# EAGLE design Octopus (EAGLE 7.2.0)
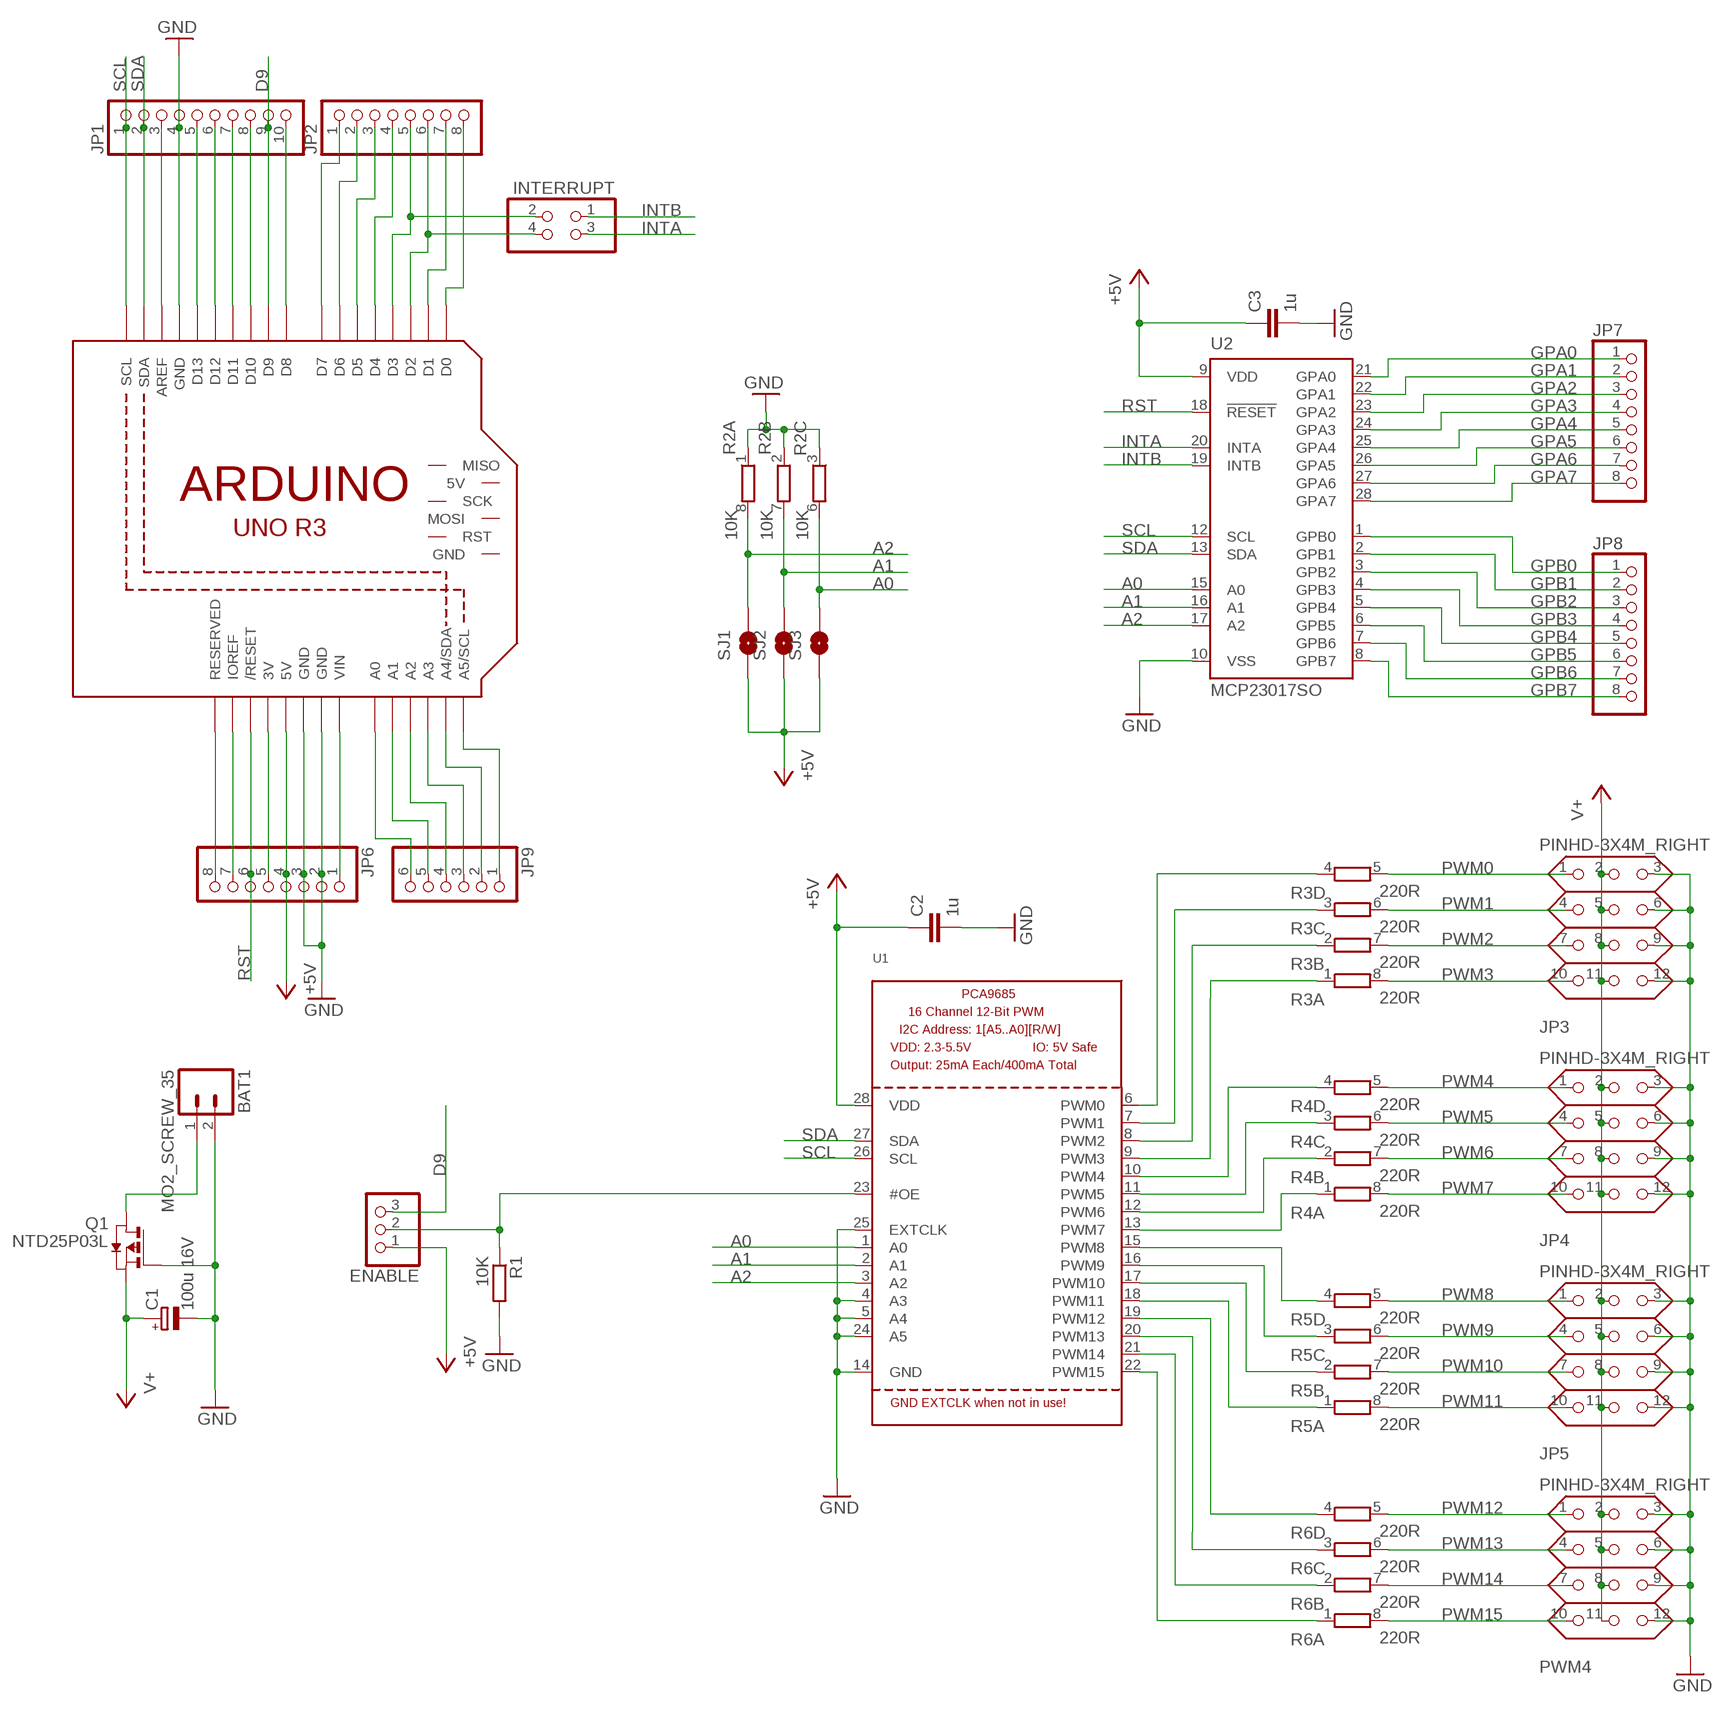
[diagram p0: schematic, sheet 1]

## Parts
BAT1  MO2_SCREW_35  [SCREWTERMINAL-3.5MM-2-NS]
C1  100u 16V  CPOLPANASONIC_E  [PANASONIC_E]
C2  1u  C0805  [C0805]
C3  1u  C0805  [C0805]
ENABLE  PINHD-1X3  [1X03M]
INTERRUPT  PINHD-2X2  [2X02M]
JP1  PINHD-1X10F_LONG  [1X10F_LONG]
JP2  PINHD-1X8F_LONG  [1X08F_LONG]
JP3  PINHD-3X4M_RIGHT  [3X04M_RIGHT]
JP4  PINHD-3X4M_RIGHT  [3X04M_RIGHT]
JP5  PINHD-3X4M_RIGHT  [3X04M_RIGHT]
JP6  PINHD-1X8F_LONG  [1X08F_LONG]
JP7  PINHD-1X81X08M_RIGHT  [1X08M_RIGHT]
JP8  PINHD-1X81X08M_RIGHT  [1X08M_RIGHT]
JP9  PINHD-1X6F_LONG  [1X06F_LONG]
M1  ARDUINO_R3_ICSP  [ARDUINOR3_ICSP]
PWM4  PINHD-3X4M_RIGHT  [3X04M_RIGHT]
Q1  NTD25P03L  [DPACK_2]
R1  10K  R0805  [R0805]
R2  10K  RESISTOR-ARRAY0603-ARV  [R0603X4]
R3  220R  RESISTOR-ARRAY0603-ARV  [R0603X4]
R4  220R  RESISTOR-ARRAY0603-ARV  [R0603X4]
R5  220R  RESISTOR-ARRAY0603-ARV  [R0603X4]
R6  220R  RESISTOR-ARRAY0603-ARV  [R0603X4]
SJ1  JUMPER-PAD-2-NOYES_SILK  [PAD-JUMPER-2-NO_YES_SILK]
SJ2  JUMPER-PAD-2-NOYES_SILK  [PAD-JUMPER-2-NO_YES_SILK]
SJ3  JUMPER-PAD-2-NOYES_SILK  [PAD-JUMPER-2-NO_YES_SILK]
U1  PCA9685  [TSSOP28]
U2  MCP23017SO  [SO28W]

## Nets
+5V: C2.1 C3.1 ENABLE.1 JP6.4 M1.5V SJ1.1 SJ2.1 SJ3.1 U1.28(VDD) U2.9(VDD)
A0: R2.6 SJ3.2 U1.1(A0) U2.15(A0)
A1: R2.7 SJ2.2 U1.2(A1) U2.16(A1)
A2: R2.8 SJ1.2 U1.3(A2) U2.17(A2)
D9: ENABLE.3 JP1.9 M1.D9
GND: BAT1.2 C1.- C2.2 C3.2 JP1.4 JP3.3 JP3.6 JP3.9 JP3.12 JP4.3 JP4.6 JP4.9 JP4.12 JP5.3 JP5.6 JP5.9 JP5.12 JP6.2 JP6.3 M1.GND M1.GND@1(GND) M1.GND@2(GND) PWM4.3 PWM4.6 PWM4.9 PWM4.12 Q1.G R1.2 R2.1 R2.2 R2.3 U1.4(A3) U1.5(A4) U1.14(GND) U1.24(A5) U1.25(EXTCLK) U2.10(VSS)
GPA0: JP7.1 U2.21(GPA0)
GPA1: JP7.2 U2.22(GPA1)
GPA2: JP7.3 U2.23(GPA2)
GPA3: JP7.4 U2.24(GPA3)
GPA4: JP7.5 U2.25(GPA4)
GPA5: JP7.6 U2.26(GPA5)
GPA6: JP7.7 U2.27(GPA6)
GPA7: JP7.8 U2.28(GPA7)
GPB0: JP8.1 U2.1(GPB0)
GPB1: JP8.2 U2.2(GPB1)
GPB2: JP8.3 U2.3(GPB2)
GPB3: JP8.4 U2.4(GPB3)
GPB4: JP8.5 U2.5(GPB4)
GPB5: JP8.6 U2.6(GPB5)
GPB6: JP8.7 U2.7(GPB6)
GPB7: JP8.8 U2.8(GPB7)
INTA: INTERRUPT.3 U2.20(INTA)
INTB: INTERRUPT.1 U2.19(INTB)
N$1: R3.4 U1.6(PWM0)
N$2: R3.3 U1.7(PWM1)
N$3: R3.2 U1.8(PWM2)
N$4: R3.1 U1.9(PWM3)
N$5: R4.4 U1.10(PWM4)
N$6: R4.3 U1.11(PWM5)
N$7: R4.2 U1.12(PWM6)
N$8: R4.1 U1.13(PWM7)
N$9: R5.4 U1.15(PWM8)
N$10: R5.3 U1.16(PWM9)
N$11: R5.2 U1.17(PWM10)
N$12: R5.1 U1.18(PWM11)
N$13: R6.4 U1.19(PWM12)
N$14: R6.3 U1.20(PWM13)
N$15: R6.2 U1.21(PWM14)
N$16: R6.1 U1.22(PWM15)
N$17: JP1.3 M1.AREF
N$18: JP1.5 M1.D13
N$19: BAT1.1 Q1.D
N$20: JP1.6 M1.D12
N$21: JP1.7 M1.D11
N$22: JP1.8 M1.D10
N$23: JP1.10 M1.D8
N$24: JP2.1 M1.D7
N$25: JP2.2 M1.D6
N$26: JP2.3 M1.D5
N$27: JP2.4 M1.D4
N$28: JP2.7 M1.D1
N$29: JP2.8 M1.D0
N$30: JP6.8 M1.RESERVED
N$31: JP6.7 M1.IOREF
N$32: JP6.5 M1.3V
N$33: JP6.1 M1.VIN
N$34: INTERRUPT.2 JP2.5 M1.D3
N$35: JP9.6 M1.A0
N$36: JP9.5 M1.A1
N$37: JP9.4 M1.A2
N$38: JP9.3 M1.A3
N$39: JP9.2 M1.A4(A4/SDA)
N$40: JP9.1 M1.A5(A5/SCL)
N$41: INTERRUPT.4 JP2.6 M1.D2
N$42: ENABLE.2 R1.1 U1.23(#OE)
PWM0: JP3.1 R3.5
PWM1: JP3.4 R3.6
PWM2: JP3.7 R3.7
PWM3: JP3.10 R3.8
PWM4: JP4.1 R4.5
PWM5: JP4.4 R4.6
PWM6: JP4.7 R4.7
PWM7: JP4.10 R4.8
PWM8: JP5.1 R5.5
PWM9: JP5.4 R5.6
PWM10: JP5.7 R5.7
PWM11: JP5.10 R5.8
PWM12: PWM4.1 R6.5
PWM13: PWM4.4 R6.6
PWM14: PWM4.7 R6.7
PWM15: PWM4.10 R6.8
RST: JP6.6 M1.RESET(/RESET) U2.18(!RESET)
SCL: JP1.1 M1.SCL U1.26(SCL) U2.12(SCL)
SDA: JP1.2 M1.SDA U1.27(SDA) U2.13(SDA)
V+: C1.+ JP3.2 JP3.5 JP3.8 JP3.11 JP4.2 JP4.5 JP4.8 JP4.11 JP5.2 JP5.5 JP5.8 JP5.11 PWM4.2 PWM4.5 PWM4.8 PWM4.11 Q1.S
Unconnected: M1.5V_ICSP(5V) M1.GND@3(GND) M1.MISO M1.MOSI M1.RESET_ICSP(RST) M1.SCK R2.4 R2.5

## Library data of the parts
BAT1 = Max-Connectors:MO2_SCREW_35
C1 = Max-RCL:CPOL
C2 C3 = Max-RCL:C
ENABLE = Max-PinHead:PINHD-1X3: PIN HEADER
INTERRUPT = Max-PinHead:PINHD-2X2
JP1 = Max-PinHead:PINHD-1X10: PIN HEADER
JP2 JP6-JP8 = Max-PinHead:PINHD-1X8: PIN HEADER
JP3-JP5 PWM4 = Max-PinHead:PINHD-3X4
JP9 = Max-PinHead:PINHD-1X6: PIN HEADER
M1 = Max-Arduino:ARDUINO_R3_ICSP
Q1 = Max-Mosfets:NTD25P03L
R1 = Max-RCL:R
R2-R6 = Max-RCL:RESISTOR-ARRAY: Array Chip Resistor Source: RS Component / Phycomp
SJ1-SJ3 = Max-Connectors:JUMPER-PAD-2-NO
U1 = Max-IOExpanders:PCA9685: PCA9685 - 16 Channel 12-Bit I2C PWM Controller 5.0V tolerant 16 channel, 12-bit I2C PWM controller with 25mA per output (max. 400mA total) Digikey: 568-5931-1-ND
U2 = Max-IOExpanders:MCP23017: http://ww1.microchip.com/downloads/en/DeviceDoc/21952a.pdf Source: http://ww1.microchip.com/downloads/en/DeviceDoc/21952a.pdf

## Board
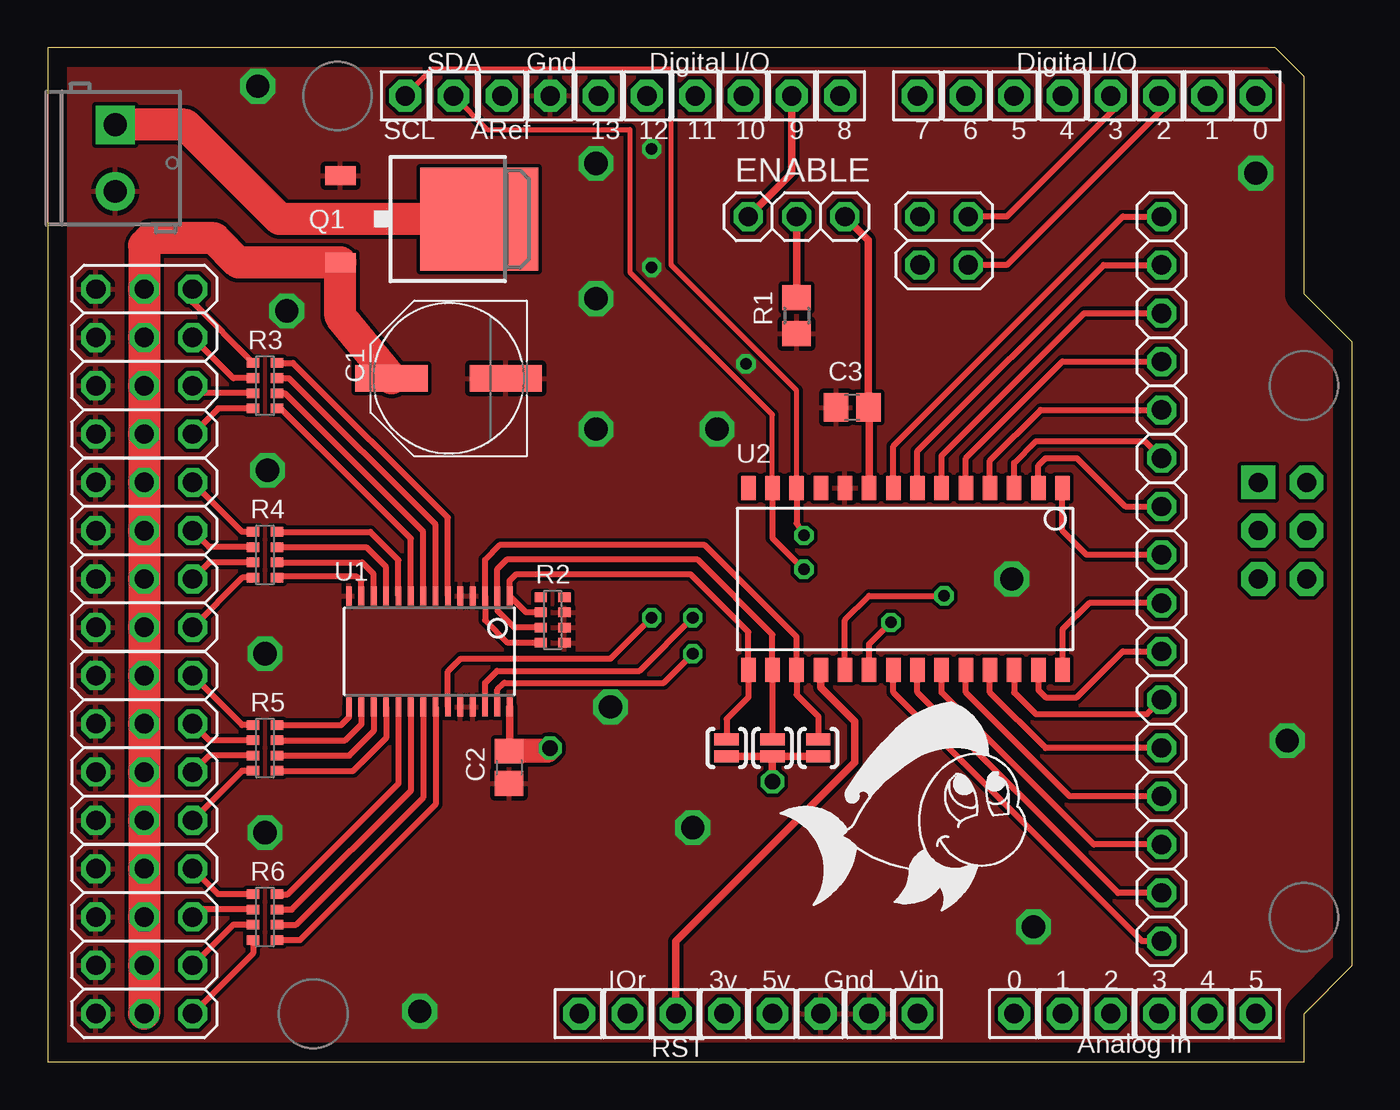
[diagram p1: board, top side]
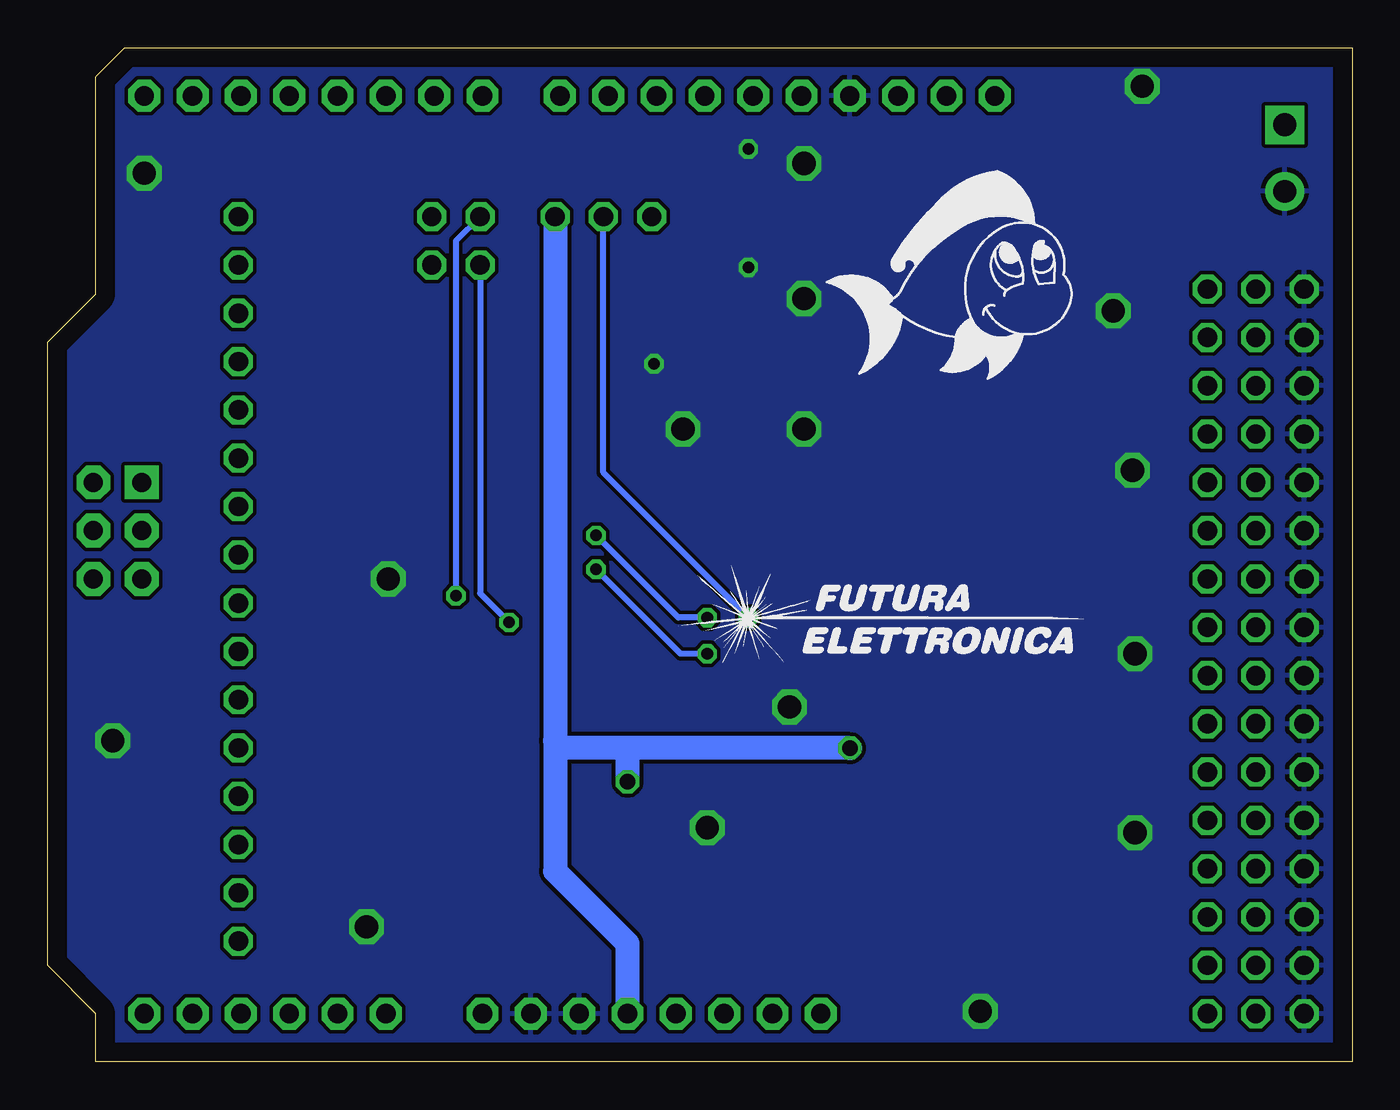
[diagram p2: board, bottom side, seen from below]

Size 68.58 x 53.34 mm. Coordinates in mm from the lower left corner, seen from the top.
Copper layers (1*16): Top 0.035mm / dielectric 1.5mm / Bottom 0.035mm
Design rules "default": minimum track width 10mil, minimum drill 24mil, track to track 8mil, track to pad 8mil, pad to pad 8mil, via to via 8mil, smd to smd 8mil, copper to edge 40mil, drill to drill 8mil, minimum pad ring 10mil, minimum via ring 8mil, stop-mask expansion 4mil, vias tented up to drill 0mil, thermal gap 10mil

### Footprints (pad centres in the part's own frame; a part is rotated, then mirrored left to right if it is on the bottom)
SCREWTERMINAL-3.5MM-2-NS = drill 1.2 pad 2.032 square: 1 -1.778,0 | drill 1.2 pad 2.032: 2 1.722,0
PANASONIC_E = smd 3.8 x 1.4: + 3,0; - -3,0
C0805 = smd 1.3 x 1.5: 1 -0.85,0; 2 0.85,0
1X03M = drill 1.016 octagon: 1 -2.54,0; 2 0,0; 3 2.54,0
2X02M = drill 1.016 octagon: 1 -1.27,-1.27; 2 -1.27,1.27; 3 1.27,-1.27; 4 1.27,1.27
1X10F_LONG = drill 1.016 octagon: 1 -11.43,0; 2 -8.89,0; 3 -6.35,0; 4 -3.81,0; 5 -1.27,0; 6 1.27,0; 7 3.81,0; 8 6.35,0; 9 8.89,0; 10 11.43,0
1X08F_LONG = drill 1.016 octagon: 1 -8.89,0; 2 -6.35,0; 3 -3.81,0; 4 -1.27,0; 5 1.27,0; 6 3.81,0; 7 6.35,0; 8 8.89,0
3X04M_RIGHT = drill 1.016 octagon: 1 -2.54,-3.81; 2 0,-3.81; 3 2.54,-3.81; 4 -2.54,-1.27; 5 0,-1.27; 6 2.54,-1.27; 7 -2.54,1.27; 8 0,1.27; 9 2.54,1.27; 10 -2.54,3.81; 11 0,3.81; 12 2.54,3.81
1X08M_RIGHT = drill 1.016 octagon: 1 -8.89,0; 2 -6.35,0; 3 -3.81,0; 4 -1.27,0; 5 1.27,0; 6 3.81,0; 7 6.35,0; 8 8.89,0
1X06F_LONG = drill 1.016 octagon: 1 -6.35,0; 2 -3.81,0; 3 -1.27,0; 4 1.27,0; 5 3.81,0; 6 6.35,0
ARDUINOR3_ICSP = drill 1 pad 1.676 octagon: 3V 35.56,2.54; 5V 38.1,2.54; A0 50.8,2.54; A1 53.34,2.54; A2 55.88,2.54; A3 58.42,2.54; A4 60.96,2.54; A5 63.5,2.54; AREF 23.876,50.8; D0 63.5,50.8; D1 60.96,50.8; D2 58.42,50.8; D3 55.88,50.8; D4 53.34,50.8; D5 50.8,50.8; D6 48.26,50.8; D7 45.72,50.8; D8 41.656,50.8; D9 39.116,50.8; D10 36.576,50.8; D11 34.036,50.8; D12 31.496,50.8; D13 28.956,50.8; GND 26.416,50.8; GND@1 43.18,2.54; GND@2 40.64,2.54; IOREF 30.48,2.54; RESERVED 27.94,2.54; RESET 33.02,2.54; SCL 18.796,50.8; SDA 21.336,50.8; VIN 45.72,2.54 | drill 1 pad 1.778 octagon: 5V_ICSP 66.167,30.48; GND@3 66.167,25.4; MOSI 66.167,27.94; RESET_ICSP 63.627,25.4; SCK 63.627,27.94 | drill 1 pad 1.778 square: MISO 63.627,30.48
DPACK_2 = smd 5.4 x 6.2: D 0,2.5 | smd 1 x 1.6: G -2.28,-4.8; S 2.28,-4.8
R0805 = smd 1.3 x 1.5: 1 -0.95,0; 2 0.95,0
R0603X4 = smd 0.5 x 0.65: 1 -1.2,-0.625; 2 -0.4,-0.625; 3 0.4,-0.625; 4 1.2,-0.625; 5 1.2,0.625; 6 0.4,0.625; 7 -0.4,0.625; 8 -1.2,0.625
PAD-JUMPER-2-NO_YES_SILK = smd 0.635 x 1.27: 1 -0.45,0; 2 0.45,0
TSSOP28 = smd 0.305 x 0.991: 1 -4.225,-2.918; 2 -3.575,-2.918; 3 -2.925,-2.918; 4 -2.275,-2.918; 5 -1.625,-2.918; 6 -0.975,-2.918; 7 -0.325,-2.918; 8 0.325,-2.918; 9 0.975,-2.918; 10 1.625,-2.918; 11 2.275,-2.918; 12 2.925,-2.918; 13 3.575,-2.918; 14 4.225,-2.918; 15 4.225,2.918; 16 3.575,2.918; 17 2.925,2.918; 18 2.275,2.918; 19 1.625,2.918; 20 0.975,2.918; 21 0.325,2.918; 22 -0.325,2.918; 23 -0.975,2.918; 24 -1.625,2.918; 25 -2.275,2.918; 26 -2.925,2.918; 27 -3.575,2.918; 28 -4.225,2.918
SO28W = smd 0.762 x 1.27: 1 -7.62,-4.78; 2 -6.35,-4.78; 3 -5.08,-4.78; 4 -3.81,-4.78; 5 -2.54,-4.78; 6 -1.27,-4.78; 7 0,-4.78; 8 1.27,-4.78; 9 2.54,-4.78; 10 3.81,-4.78; 11 5.08,-4.78; 12 6.35,-4.78; 13 7.62,-4.78; 14 8.89,-4.78; 15 8.89,4.78; 16 7.62,4.78; 17 6.35,4.78; 18 5.08,4.78; 19 3.81,4.78; 20 2.54,4.78; 21 1.27,4.78; 22 0,4.78; 23 -1.27,4.78; 24 -2.54,4.78; 25 -3.81,4.78; 26 -5.08,4.78; 27 -6.35,4.78; 28 -7.62,4.78

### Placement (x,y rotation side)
BAT1  3.56,47.5 270 top
C1  21.08,35.94 180 top
C2  24.26,15.49 270 top
C3  42.29,34.42 180 top
ENABLE  39.37,44.45 180 top
INTERRUPT  47.12,43.18 270 top
JP1  30.23,50.8 0 top
JP2  54.61,50.8 0 top
JP3  5.08,36.83 180 top
JP4  5.08,26.67 180 top
JP5  5.08,16.51 180 top
JP6  36.83,2.54 180 top
JP7  58.55,15.24 90 top
JP8  58.55,35.56 90 top
JP9  57.15,2.54 180 top
M1  0,0 0 top
PWM4  5.08,6.35 180 top
Q1  20.19,44.32 270 top
R1  39.37,39.24 270 top
R2  26.54,23.24 90 top
R3  11.43,35.56 90 top
R4  11.43,26.67 90 top
R5  11.43,16.51 90 top
R6  11.43,7.62 90 top
SJ1  40.51,16.51 90 top
SJ2  38.1,16.51 90 top
SJ3  35.69,16.51 90 top
U1  20.07,21.59 180 top
U2  45.72,25.4 180 top
U$1  [FISHINO]  40.26,8.26 0 top
U$2  [FISHINO]  25.91,36.2 0 bottom
U$4  [FUTURA]  35.43,20.95 0 bottom

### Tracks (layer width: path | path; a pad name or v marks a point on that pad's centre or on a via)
+5V  (via drill 0.81)
  Top 0.406: U1.28 24.29,16.38 C2.1 | U2.9 43.18,34.38 C3.1 43.14,43.22 ENABLE.1 | SJ2.1 SJ1.1 | SJ3.1 SJ2.1 | SJ2.1 v38.1,14.73
  Top 1.27: 24.29,16.38 26.28,16.38 v26.42,16.51
  Bottom 1.27: JP6.4 38.1,6.22 41.91,10.03 41.91,16.89 | v26.42,16.51 38.1,16.51 | 38.1,16.51 41.53,16.51 41.91,16.89 | ENABLE.1 41.91,16.89 | v38.1,14.73 38.1,16.51
A0
  Top 0.305: SJ3.2 35.69,18.03 36.83,19.18 U2.15 36.83,22.61 33.78,25.65 24.64,25.65 24.29,25.31 U1.1 25.16,23.64 R2.6
A1
  Top 0.305: R2.7 24.53,22.84 23.64,23.73 U1.2 23.64,25.93 24.13,26.42 34.16,26.42 38.1,22.48 U2.16 SJ2.2
A2
  Top 0.305: R2.8 24.19,22.04 22.99,23.24 U1.3 22.99,26.42 23.75,27.18 34.54,27.18 39.37,22.35 U2.17 39.37,19.3 40.51,18.16 SJ1.2
D9
  Top 0.406: ENABLE.3 39.12,46.74 JP1.9
GND  (via drill 0.61, 1.22)
  other vias: 11.43,12.06 11.43,21.46 11.56,31.11 12.57,39.5 35.18,33.27 28.83,33.27 19.56,2.67 33.91,12.32 29.59,18.67 50.67,25.4 28.83,47.24 28.83,40.13 11.05,51.31 51.82,7.11 65.15,16.89 63.5,46.74 31.75,41.78 31.75,48.01 36.7,36.7
  pour Top: 0,0 68.71,0 68.58,53.34 -0.13,53.34
  pour Bottom: 0,0 68.71,0 68.58,53.34 -0.13,53.34
GPA0
  Top 0.305: JP7.1 57.53,6.35 44.45,19.43 U2.21
GPA1
  Top 0.305: JP7.2 56.26,8.89 45.72,19.43 U2.22
GPA2
  Top 0.305: JP7.3 54.99,11.43 46.99,19.43 U2.23
GPA3
  Top 0.305: JP7.4 53.72,13.97 48.26,19.43 U2.24
GPA4
  Top 0.305: JP7.5 52.45,16.51 49.53,19.43 U2.25
GPA5
  Top 0.305: U2.26 50.8,19.43 51.94,18.29 57.78,18.29 JP7.6
GPA6
  Top 0.305: U2.27 52.07,19.56 52.45,19.18 54.1,19.18 56.52,21.59 JP7.7
GPA7
  Top 0.305: JP7.8 54.74,24.13 53.34,22.73 U2.28
GPB0
  Top 0.305: JP8.1 54.61,26.67 53.34,27.94 U2.1
GPB1
  Top 0.305: U2.2 52.07,31.37 52.45,31.75 54.1,31.75 56.64,29.21 JP8.2
GPB2
  Top 0.305: U2.3 50.8,31.5 51.94,32.64 57.66,32.64 JP8.3
GPB3
  Top 0.305: U2.4 49.53,31.62 52.2,34.29 JP8.4
GPB4
  Top 0.305: U2.5 48.26,31.75 53.34,36.83 JP8.5
GPB5
  Top 0.305: U2.6 46.99,31.88 54.48,39.37 JP8.6
GPB6
  Top 0.305: U2.7 45.72,32.13 55.5,41.91 JP8.7
GPB7
  Top 0.305: U2.8 44.45,32.38 56.52,44.45 JP8.8
INTA  (via drill 0.61)
  Top 0.305: U2.20 43.18,21.97 v44.32,23.11
  Bottom 0.305: INTERRUPT.3 45.85,24.64 v44.32,23.11
INTB  (via drill 0.61)
  Top 0.305: U2.19 41.91,23.24 43.18,24.51 v47.12,24.51
  Bottom 0.305: INTERRUPT.1 47.12,43.18 v47.12,24.51
N$1
  Top 0.305: U1.6 21.04,28.62 12.9,36.76 R3.4
N$2
  Top 0.305: U1.7 20.39,28.25 12.68,35.96 R3.3
N$3
  Top 0.305: U1.8 19.74,27.88 12.46,35.16 R3.2
N$4
  Top 0.305: U1.9 19.09,27.52 12.25,34.36 R3.1
N$5
  Top 0.305: U1.10 18.44,26.39 16.96,27.87 R4.4
N$6
  Top 0.305: U1.11 17.79,26.02 16.75,27.07 R4.3
N$7
  Top 0.305: U1.12 17.14,25.66 16.53,26.27 R4.2
N$8
  Top 0.254: 12.11,25.53 R4.1
  Top 0.305: U1.13 16.49,25.29 16.26,25.53 12.11,25.53
N$9
  Top 0.305: U1.15 15.84,18.13 15.42,17.71 R5.4
N$10
  Top 0.305: R5.3 15.64,16.91 16.49,17.76 U1.16
N$11
  Top 0.305: U1.17 17.14,17.39 15.86,16.11 R5.2
N$12
  Top 0.305: R5.1 16.07,15.31 17.79,17.03 U1.18
N$13
  Top 0.305: U1.19 18.44,14.63 12.63,8.82 R6.4
N$14
  Top 0.305: U1.20 19.09,14.27 12.85,8.02 R6.3
N$15
  Top 0.305: U1.21 19.74,13.9 13.06,7.22 R6.2
N$16
  Top 0.305: U1.22 20.39,13.53 13.28,6.42 R6.1
N$19
  Top 1.676: BAT1.1 7.24,49.28 12.19,44.32 Q1.D
N$34
  Top 0.305: JP2.5 56.01,50.04 50.42,44.45 INTERRUPT.2
N$41
  Top 0.305: JP2.6 58.55,50.04 50.42,41.91 INTERRUPT.4
N$42  (via drill 0.61)
  Top 0.305: U1.23 21.04,20.53 21.72,21.21 29.59,21.21 v31.75,23.37
  Top 0.406: R1.1 ENABLE.2
  Bottom 0.305: v31.75,23.37 39.37,30.99 ENABLE.2
PWM0
  Top 0.305: JP3.1 7.62,39.95 R3.5
PWM1
  Top 0.305: R3.6 9.76,35.96 JP3.4
PWM2
  Top 0.305: R3.7 8.02,35.16 JP3.7
PWM3
  Top 0.305: R3.8 8.96,34.36 JP3.10
PWM4
  Top 0.305: R4.5 10.23,27.87 JP4.1
PWM5
  Top 0.305: R4.6 8.49,27.07 JP4.4
PWM6
  Top 0.305: R4.7 8.49,26.27 JP4.7
PWM7
  Top 0.305: R4.8 10.23,25.47 JP4.10
PWM8
  Top 0.305: R5.5 10.23,17.71 JP5.1
PWM9
  Top 0.305: R5.6 8.49,16.91 JP5.4
PWM10
  Top 0.305: R5.7 8.49,16.11 JP5.7
PWM11
  Top 0.305: R5.8 10.23,15.31 JP5.10
PWM12
  Top 0.305: R6.5 8.96,8.82 PWM4.1
PWM13
  Top 0.305: R6.6 8.02,8.02 PWM4.4
PWM14
  Top 0.305: R6.7 9.76,7.22 PWM4.7
PWM15
  Top 0.305: R6.8 10.8,5.72 PWM4.10
RST
  Top 0.406: U2.18 40.64,19.68 42.42,17.91 42.42,15.75 33.02,6.35 JP6.6
SCL  (via drill 0.61)
  Top 0.254: JP1.1 20.19,52.2 32.77,52.2 32.77,41.91 39.37,35.31 U2.12
  Top 0.305: U1.26 22.99,19.94 23.62,20.57 31.11,20.57 v33.91,23.37 | U2.12 39.37,28.32 v39.75,27.69
  Bottom 0.305: v33.91,23.37 35.43,23.37 v39.75,27.69
SDA  (via drill 0.61)
  Top 0.254: U2.13 38.1,34.04 30.61,41.53 30.61,49.02 23.11,49.02 JP1.2
  Top 0.305: U1.27 23.64,19.58 24,19.94 32.38,19.94 v33.91,21.46 | U2.13 38.1,27.56 v39.75,25.91
  Bottom 0.305: v33.91,21.46 35.31,21.46 v39.75,25.91
V+
  Top 1.676: PWM4.11 PWM4.8 PWM4.5 PWM4.2 JP5.11 JP5.8 JP5.5 JP5.2 JP4.11 JP4.8 JP4.5 JP4.2 JP3.11 JP3.8 JP3.5 JP3.2 5.08,42.93 5.46,43.31 8.76,43.31 10.03,42.04 Q1.S 15.39,39.23 C1.+

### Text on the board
tDocu: + | V+ | INTB=D3 | - | B7 | GND | V+ | PWM | D9 | OFF | B6 | 0 | INTA=D2 | B5 | 1 | B4 | 2 | B3 | 3 | B2 | 4 | B1 | 5 | DESIGNED BY / MASSIMO DEL FEDELE | B0 | 6 | PCA9685 | 7 | A7 | A6 | 8 | 9 | I2C ADDRESS | A5 | PWM/SERVO | A4 | 10 | A0 | A1 | A2 | A3 | 11 | FISHINO | A2 | 12 | OCTOPUS | A1 | 13 | DIGITAL I/O | A0 | PWM AND DIGITAL I/O EXPANDER | 14 | 15
bDocu: B7 | GND | V+ | PWM | 0 | B6 | B5 | 1 | B4 | 2 | B3 | 3 | www.fishino.com | B2 | 4 | FISHINO OCTOPUS | B1 | 5 | B0 | 6 | 7 | A7 | A6 | 8 | 9 | A5 | A4 | 10 | A3 | 11 | A2 | PWM AND DIGITAL I/O EXPANDER | 12 | DESIGNED BY MASSIMO DEL FEDELE | A1 | 13 | A0 | 14 | 15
